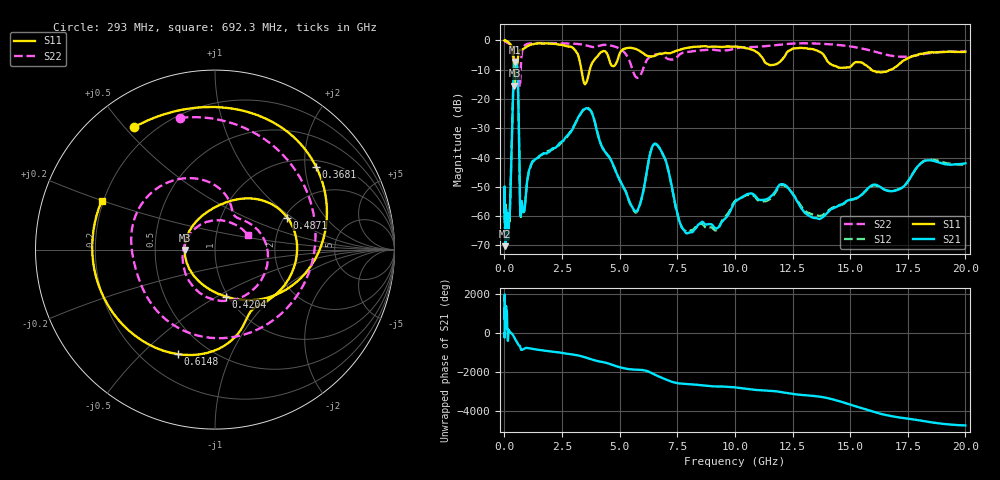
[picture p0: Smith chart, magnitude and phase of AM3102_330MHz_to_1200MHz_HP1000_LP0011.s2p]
! Date/Time: Tue, Sep 11, 2018 5:16 PM
! Network Analyzer: Agilent Technologies E8362B Rev: A.07.50.63
! Sweep from 0.010 to 20.000 GHz, 1601 Points, Sweep Type: LOG
! Power Supply: 4.949 V, 0.001 A
# Hz S DB R 50
!freq MagS11 AngS11 MagS21 AngS21 MagS12 AngS12 MagS22 AngS22
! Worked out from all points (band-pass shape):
!   1601 points, 10 MHz to 20 GHz, reference 50 ohm
!   highest |S21| = -7.32 dB at 458 MHz (marker M1); lowest = -70.3 dB at 43.2 MHz (marker M2)
!   |S21| within 3 dB of the highest: 411.6 MHz to 566.4 MHz (154.8 MHz wide, 31.7 % of centre)
!   lowest |S11| = -15.4 dB at 438.8 MHz (marker M3), VSWR 1.41, Z = 35.5 - j0.201 ohm
!   |S11| at or under -10 dB: 416.6 MHz to 465.1 MHz (48.48 MHz wide, 11 % of centre); 3.341 GHz to 3.702 GHz (361.1 MHz wide, 10.3 % of centre); 15.91 GHz to 16.76 GHz (850.6 MHz wide, 5.21 % of centre)
!   |S22| runs from -15.9 to -0.2 dB; largest |S21 - S12| = 0.0052
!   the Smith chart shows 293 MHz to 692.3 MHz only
!   S11 on the Smith chart (normalised r, x): 293 MHz: 0.13, +0.53; 368.1 MHz: 1.17, +2.29; 420.4 MHz: 0.97, -0.55; 487.1 MHz: 2.07, +0.92; 614.8 MHz: 0.34, -0.65; 692.3 MHz: 0.19, +0.20
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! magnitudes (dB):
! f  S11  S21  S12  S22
! 10 MHz  0.0  -53.1  -51.0  -0.2
! 35.55 MHz  0.0  -63.7  -62.1  -0.3
! 43.2 MHz  0.0  -70.3  -66.8  -0.4
! 48.64 MHz  0.0  -59.3  -56.5  -0.4
! 126.4 MHz  -0.4  -65.4  -64.8  -0.8
! 222.5 MHz  -1.1  -60.3  -61.9  -1.3
! 293 MHz  -1.7  -43.0  -43.2  -2.4
! 368.1 MHz  -2.8  -20.4  -20.5  -5.5
! 420.4 MHz  -11.4  -9.1  -9.2  -6.6
! 438.8 MHz  -15.4  -7.7  -7.7  -6.9
! 447.2 MHz  -14.8  -7.4  -7.5  -6.8
! 458 MHz  -12.0  -7.3  -7.4  -6.6
! 487.1 MHz  -7.1  -7.6  -7.6  -6.4
! 614.8 MHz  -4.2  -24.1  -24.1  -10.2
! 692.3 MHz  -3.3  -58.7  -58.9  -13.9
! 1.59 GHz  -1.0  -39.1  -39.1  -0.9
! 3.634 GHz  -12.4  -23.3  -23.1  -1.9
! 5.652 GHz  -2.8  -58.2  -58.5  -11.9
! 6.549 GHz  -5.2  -35.3  -35.5  -4.8
! 7.995 GHz  -2.4  -65.8  -65.2  -3.9
! 13.68 GHz  -3.9  -61.0  -60.0  -1.1
! 20 GHz  -3.9  -42.0  -42.5  -3.8
